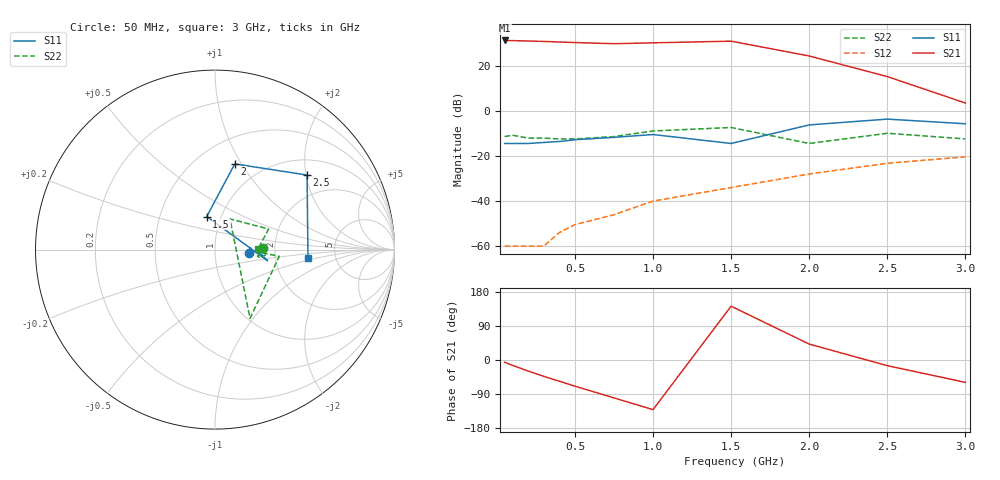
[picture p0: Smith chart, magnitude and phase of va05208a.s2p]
!  IVA-05208  S PARAMETERS
!  Full Gain S PARAMETERS (VGC=0)  LAST UPDATED 08-11-93
# ghz s ma r 50
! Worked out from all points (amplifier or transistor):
!   12 points, 50 MHz to 3 GHz, reference 50 ohm
!   highest |S21| = 31.3 dB at 50 MHz (marker M1)
!   |S21| within 3 dB of that: start of sweep to 1.704 GHz
!   unconditionally stable (mu >= 1): start of sweep to 1.374 GHz; 2.627 GHz to end of sweep
!   at 200 MHz: K = 12.65, MAG = 31.5 dB, |S12| = -60.0 dB
!   at 750 MHz: K = 2.81, MAG = 30.6 dB, |S12| = -46.0 dB
!   at 3 GHz: K = 2.36, MAG = 5.4 dB, |S12| = -20.4 dB
!   S11 on the Smith chart (normalised r, x): 50 MHz: 1.47, -0.05; 1.5 GHz: 0.85, +0.33; 2 GHz: 0.75, +0.94; 2.5 GHz: 1.38, +2.03; 3 GHz: 3.11, -0.39
0.05  0.19 -5.0  36.7 -6.0  0.001 62.0  0.27 2.0
0.1  0.19 -3.0  36.4 -14.0  0.001 58.0  0.29 -5.0
0.2  0.19 0.0  35.7 -29.0  0.001 76.0  0.25 -11.0
0.3  0.2 2.0  34.9 -43.0  0.001 103.0  0.25 -10.0
0.4  0.21 -2.0  33.9 -56.0  0.002 114.0  0.24 -9.0
0.5  0.23 -3.0  33 -69.0  0.003 115.0  0.24 -8.0
0.75  0.26 -6.0  31.1 -100.0  0.005 132.0  0.27 -4.0
1  0.3 -12.0  32.5 -131.0  0.01 133.0  0.36 -6.0
1.5  0.19 104.0  35.4 142.0  0.02 124.0  0.43 -63.0
2  0.49 77.0  16.6 42.0  0.04 123.0  0.19 64.0
2.5  0.66 39.0  5.8 -15.0  0.069 114.0  0.32 21.0
3  0.52 -5.0  1.5 -59.0  0.096 95.0  0.24 1.0
